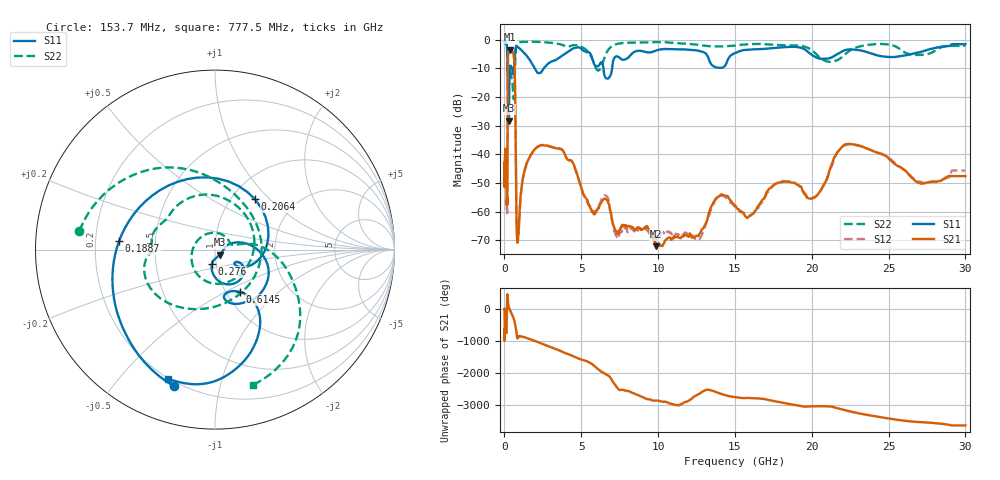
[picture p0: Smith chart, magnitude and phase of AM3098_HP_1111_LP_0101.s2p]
! Date/Time: Thu, Feb 28, 2019 8:47 AM
! Network Analyzer: Agilent Technologies E8364B Rev: A.07.50.67
! Sweep from 0.010 to 30.000 GHz, 1601 Points, Sweep Type: LOG
! Power Supply: 5.022 V, 0.001 A
# Hz S DB R 50
!freq MagS11 AngS11 MagS21 AngS21 MagS12 AngS12 MagS22 AngS22
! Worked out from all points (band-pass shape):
!   1601 points, 10 MHz to 30 GHz, reference 50 ohm
!   highest |S21| = -3.40 dB at 335.4 MHz (marker M1); lowest = -72.0 dB at 9.878 GHz (marker M2)
!   |S21| within 3 dB of the highest: 228.2 MHz to 624.1 MHz (395.9 MHz wide, 92.9 % of centre)
!   lowest |S11| = -28.2 dB at 288.7 MHz (marker M3), VSWR 1.08, Z = 52.7 - j2.93 ohm
!   |S11| at or under -10 dB: 210 MHz to 355.3 MHz (145.3 MHz wide, 51.4 % of centre); 1.974 GHz to 2.551 GHz (577.2 MHz wide, 25.5 % of centre); 6.439 GHz to 7.005 GHz (566.3 MHz wide, 8.42 % of centre)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
!   |S22| runs from -20.8 to -0.5 dB; largest |S21 - S12| = 0.012
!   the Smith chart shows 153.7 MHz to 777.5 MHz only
!   S11 on the Smith chart (normalised r, x): 153.7 MHz: 0.18, -0.73; 188.7 MHz: 0.30, +0.04; 206.4 MHz: 1.28, +0.82; 276 MHz: 0.95, -0.15; 614.5 MHz: 1.16, -0.59; 777.5 MHz: 0.20, -0.68
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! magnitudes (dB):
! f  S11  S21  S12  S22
! 10 MHz  -0.4  -43.5  -43.1  -0.5
! 38.04 MHz  -0.2  -41.0  -41.1  -0.6
! 92.7 MHz  -0.8  -38.9  -39.2  -1.2
! 144.7 MHz  -1.6  -55.2  -53.9  -2.0
! 153.7 MHz  -2.0  -57.3  -58.8  -2.4
! 188.7 MHz  -5.4  -53.5  -55.0  -9.2
! 206.4 MHz  -8.9  -21.8  -21.8  -9.1
! 276 MHz  -21.7  -3.8  -3.8  -9.3
! 288.7 MHz  -28.2  -3.6  -3.6  -9.6
! 335.4 MHz  -11.7  -3.4  -3.4  -9.8
! 550.5 MHz  -11.4  -4.3  -4.3  -17.6
! 614.5 MHz  -11.2  -5.9  -5.8  -20.8
! 689.5 MHz  -4.8  -16.1  -16.1  -9.3
! 777.5 MHz  -2.3  -61.5  -61.4  -2.1
! 859.3 MHz  -2.5  -69.7  -65.3  -1.2
! 2.084 GHz  -11.1  -37.7  -37.6  -0.7
! 3.76 GHz  -5.5  -38.4  -38.4  -1.8
! 7.926 GHz  -6.7  -65.4  -66.0  -1.0
! 9.878 GHz  -3.7  -72.0  -69.6  -0.8
! 20.1 GHz  -5.6  -55.1  -55.3  -4.1
! 22.56 GHz  -3.4  -36.4  -36.6  -3.5
! 30 GHz  -1.6  -47.6  -45.6  -2.1
